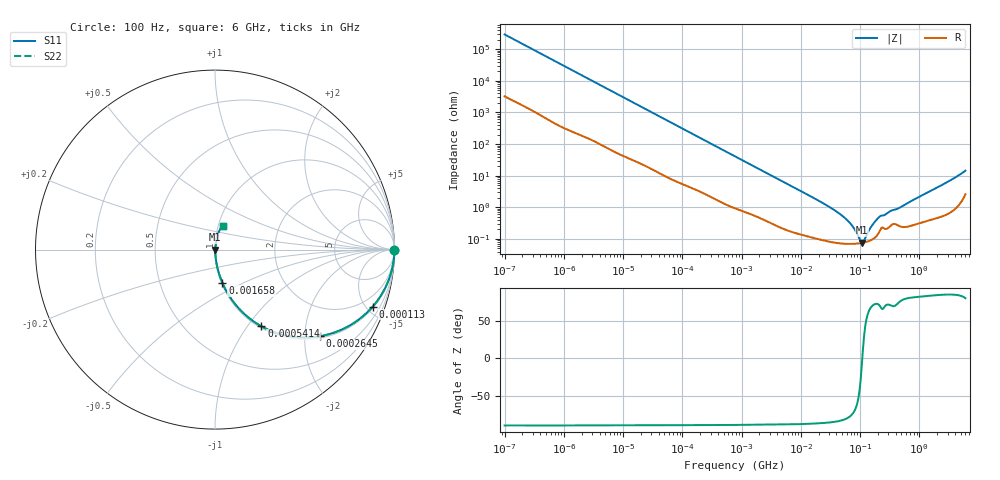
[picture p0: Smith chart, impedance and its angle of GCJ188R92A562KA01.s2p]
!Murata Part Number: GCJ188R92A562KA01
!These Parameters are Measured in Series Mode Connection
!Data Generated on Mar 13, 2026
!  o--ll--o
!Port1  Port2
!  o------o
!Operation Temp=25[degC], DC Bias Voltage=0[V]
!Freq. Start=100[Hz] Stop=6[GHz] 401[Steps]
# Hz S RI R 50
!Freq.(Hz) S11(Real) S11(Imag) S21(Real) S21(Imag) S12(Real) S12(Imag) S22(Real) S22(Imag)
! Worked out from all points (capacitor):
!   401 points, 100 Hz to 6 GHz, reference 50 ohm
!   read as one part in series: C = 5.43 nF near 109 Hz
!   lowest |Z| = 75.9 mohm at 106.7 MHz (marker M1)
!   series resonance near 109.2 MHz, so ESL is about 390 pH
!   S11 on the Smith chart (normalised r, x): 100 Hz: open; 113 kHz: 1.10, -5.48; 264.5 kHz: 1.05, -2.37; 541.4 kHz: 1.02, -1.17; 1.658 MHz: 1.01, -0.39; 6 GHz: 1.05, +0.28
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100  1 -0.000342  3.9e-06 0.000342  3.9e-06 0.000342  1 -0.000342
2008  0.9999 -0.00673  0.000129 0.00673  0.000129 0.00673  0.9999 -0.00673
12592  0.9977 -0.0414  0.00232 0.0414  0.00232 0.0414  0.9977 -0.0414
40335  0.981 -0.1287  0.019 0.1287  0.019 0.1287  0.981 -0.1287
112960  0.8782 -0.3181  0.1218 0.3181  0.1218 0.3181  0.8782 -0.3181
264476  0.5822 -0.4831  0.4178 0.4831  0.4178 0.4831  0.5822 -0.4831
541393  0.2585 -0.4274  0.7415 0.4274  0.7415 0.4274  0.2585 -0.4274
774597  0.1492 -0.3451  0.8508 0.3451  0.8508 0.3451  0.1492 -0.3451
1658239  0.0409 -0.1846  0.9591 0.1846  0.9591 0.1846  0.0409 -0.1846
4246196  0.00821 -0.0759  0.9918 0.0759  0.9918 0.0759  0.00821 -0.0759
1.555665e7  0.00154 -0.0209  0.9985 0.0209  0.9985 0.0209  0.00154 -0.0209
3.330331e7  0.000875 -0.00918  0.9991 0.00918  0.9991 0.00918  0.000875 -0.00918
5.449875e7  0.000726 -0.00468  0.9993 0.00468  0.9993 0.00468  0.000726 -0.00468
7.455971e7  0.000703 -0.00244  0.9993 0.00244  0.9993 0.00244  0.000703 -0.00244
1.066761e8  0.000745 -0.000144  0.9993 0.000144  0.9993 0.000144  0.000745 -0.000144
1.166697e8  0.00077 0.000421  0.9992 -0.000421  0.9992 -0.000421  0.00077 0.000421
1.526266e8  0.000915 0.00219  0.9991 -0.00219  0.9991 -0.00219  0.000915 0.00219
1.996653e8  0.00141 0.00424  0.9986 -0.00424  0.9986 -0.00424  0.00141 0.00424
3.124326e8  0.00244 0.00687  0.9976 -0.00687  0.9976 -0.00687  0.00244 0.00687
4.674818e8  0.0026 0.00937  0.9974 -0.00937  0.9974 -0.00937  0.0026 0.00937
2.240541e9  0.00702 0.0464  0.993 -0.0464  0.993 -0.0464  0.00702 0.0464
6e9  0.0434 0.1323  0.9566 -0.1323  0.9566 -0.1323  0.0434 0.1323
